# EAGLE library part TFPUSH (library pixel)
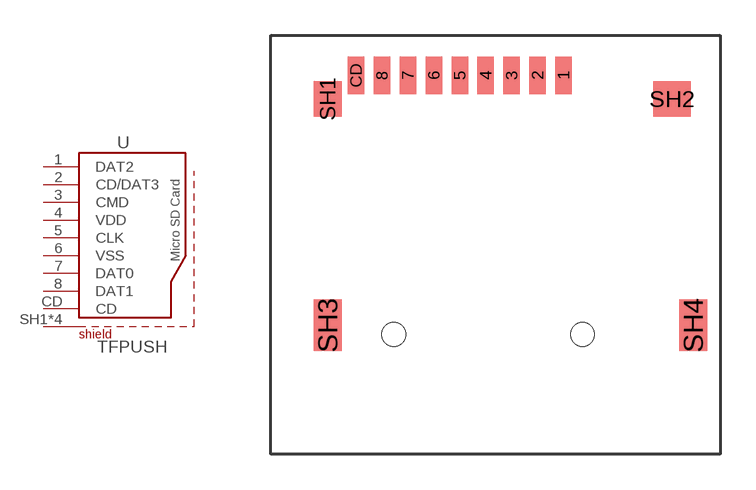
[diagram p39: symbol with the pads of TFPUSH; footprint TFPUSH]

Designator prefix -

## TFPUSH  [TFPUSH]
1  DAT2
2  CD/DAT3
3  CMD
4  VDD
5  CLK
6  VSS
7  DAT0
8  DAT1
CD  CD
SH1  SHIELD
SH2  SHIELD
SH3  SHIELD
SH4  SHIELD

## Footprint TFPUSH (pad centres in mm)
smd 0.7 x 1.6: 1 2.25,11; 2 1.15,11; 3 0.05,11; 4 -1.05,11; 5 -2.15,11; 6 -3.25,11; 7 -4.35,11; 8 -5.45,11; CD -6.55,11
smd 1.2 x 1.5: SH1 -7.75,10
smd 1.6 x 1.5: SH2 6.85,10
smd 1.2 x 2.2: SH3 -7.75,0.4; SH4 7.75,0.4
hole 1 at -4.95,0
hole 1 at 3.05,0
